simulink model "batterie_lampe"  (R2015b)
settings: Solver=VariableStepAuto  StartTime=0.0  StopTime=96000  RelTol=1e-3
libraries: fl_lib x4, nesl_utility x3, elec_lib x2, powerlib_meascontrol x1

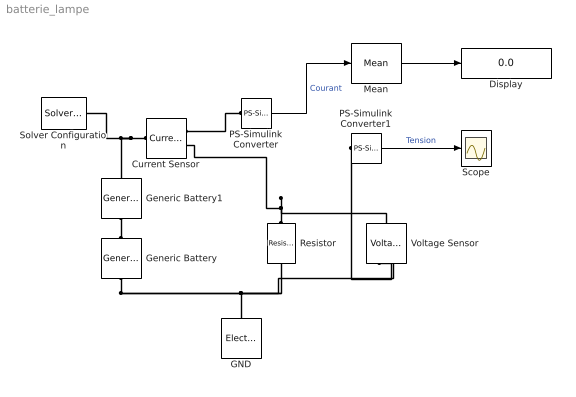
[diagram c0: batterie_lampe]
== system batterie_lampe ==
  Current Sensor : fl_lib/Electrical/Electrical Sensors/Current Sensor
  Display : Display
  GND : fl_lib/Electrical/Electrical Elements/Electrical Reference
  Generic Battery : elec_lib/Sources/Generic Battery  Vnom=14.5 V  R1=0.0058 Ohm  prm_AH=2  AH=83 hr*A  AH0=83 hr*A  V1=11.5 V  AH1=4 hr*A  prm_R2=1  R2=2e+3 Ohm
  Generic Battery1 : elec_lib/Sources/Generic Battery  Vnom=14.5 V  R1=0.0058 Ohm  prm_AH=2  AH=83 hr*A  AH0=83 hr*A  V1=11.5 V  AH1=4 hr*A  prm_R2=1  R2=2e+3 Ohm
  Mean : powerlib_meascontrol/Measurements/Mean  Freq=1/96000  Vinit=0  Ts=0
  PS-Simulink Converter : nesl_utility/PS-Simulink Converter  PhysicalDomain=network_engine_domain  SubClassName=ps_output  LeftPortType=input  RightPortType=output  PseudoPeriodic=off  Frequencies=[]  Unit=1  AffineConversion=off
  PS-Simulink Converter1 : nesl_utility/PS-Simulink Converter  PhysicalDomain=network_engine_domain  SubClassName=ps_output  LeftPortType=input  RightPortType=output  PseudoPeriodic=off  Frequencies=[]  Unit=1  AffineConversion=off
  Resistor : fl_lib/Electrical/Electrical Elements/Resistor  R=28/3 Ohm  i_specify=off  i_priority=None  i=0 A  v_specify=off  v_priority=None  v=0 V
  Scope : Scope
  Solver Configuration : nesl_utility/Solver Configuration  PhysicalDomain=network_engine_domain  SubClassName=solver  LeftPortType=input  RightPortType=generic  Accelerate=off  Tones=[]  Harmonics=[]  SimulateNoise=off  Profile=off  UseLocalSampling=off  EnableSwitchedLinearOptims=on  FrequencyDomain=off  UseCCode=off  RelTol=0.001  AbsTol=1e-06  MinStep=1e-09  ToWorkspace=off  RevertToSquareIcSolve=off  NumHomotopyIterations=100  PhasorMode=off  PhasorModeNumHarmonics=1  DoDC=off  ResidualTolerance=1e-9  UseLocalSolver=off  LocalSolverChoice=NE_TRAPEZOIDAL_ADVANCER  LocalSolverSampleTime=.001  DoFixedCost=off  MaxNonlinIter=3  MaxModeIter=2  LinearAlgebra=Sparse  DelaysMemoryBudget=1024  AutomaticFiltering=on  FilteringTimeConstant=0.001
  Voltage Sensor : fl_lib/Electrical/Electrical Sensors/Voltage Sensor
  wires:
  PS-Simulink Converter/1 -> Mean/1  "Courant"
  PS-Simulink Converter1/1 -> Scope/1  "Tension"
  Mean/1 -> Display/1
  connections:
  Resistor/LConn1 -- Current Sensor/RConn2 -- Voltage Sensor/LConn1
  Current Sensor/LConn1 -- Solver Configuration/RConn1 -- Generic Battery1/LConn1
  Generic Battery/RConn1 -- GND/LConn1 -- Voltage Sensor/RConn2 -- Resistor/RConn1
  Generic Battery/LConn1 -- Generic Battery1/RConn1
  PS-Simulink Converter/LConn1 -- Current Sensor/RConn1
  PS-Simulink Converter1/LConn1 -- Voltage Sensor/RConn1
